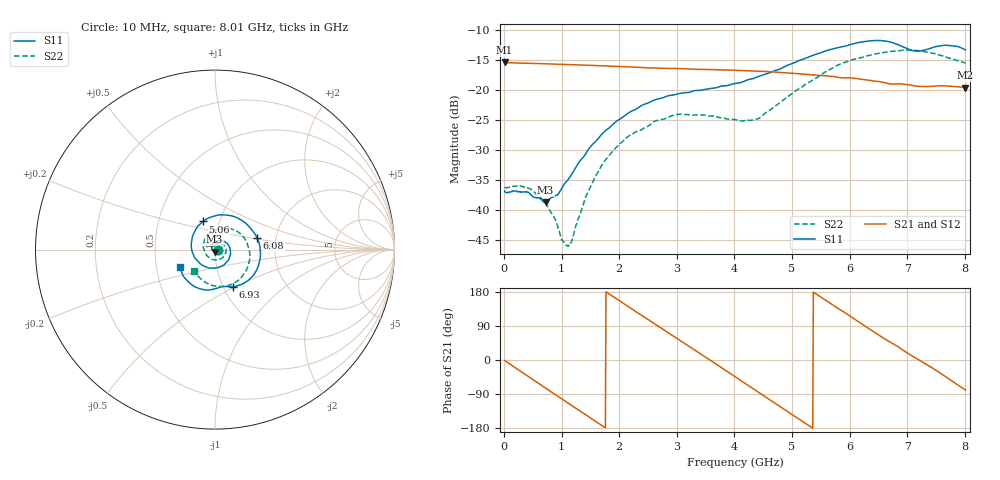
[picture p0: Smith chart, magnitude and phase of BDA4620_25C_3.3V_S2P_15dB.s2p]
!Agilent Technologies,E5071B,MY42404982,A.09.10
!Date: Wed May 06 08:51:47 2026
!Data & Calibration Information:
!Freq	S11:SOLT2(ON)	S21:SOLT2(ON)	S12:SOLT2(ON)	S22:SOLT2(ON)
# Hz S RI R 50
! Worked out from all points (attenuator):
!   801 points, 10 MHz to 8.01 GHz, reference 50 ohm
!   highest |S21| = -15.42 dB at 10 MHz (marker M1); lowest = -19.6 dB at 8.01 GHz (marker M2)
!   lowest |S11| = -38.7 dB at 720 MHz (marker M3), VSWR 1.02, Z = 49.8 - j1.13 ohm
!   |S11| at or under -10 dB: start of sweep to end of sweep
!   |S22| runs from -46.0 to -13.4 dB; largest |S21 - S12| = 0.00071
!   S11 on the Smith chart (normalised r, x): 10 MHz: 1.03, -0.00; 5.06 GHz: 0.84, +0.27; 6.08 GHz: 1.59, +0.22; 6.93 GHz: 1.11, -0.48; 8.01 GHz: 0.67, -0.13
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1e7  0.0144 -0.000941  0.1694 -0.00362  0.1696 -0.00361  0.0154 -0.000668
4.4e8  0.00887 -0.0107  0.117 -0.1188  0.1171 -0.1189  0.0135 -0.00689
7.2e8  -0.00236 -0.0114  0.0456 -0.1588  0.0456 -0.1591  0.00692 -0.00918
1.09e9  -0.0174 0.000862  -0.06 -0.1517  -0.0601 -0.1518  -0.00399 -0.0031
1.17e9  -0.0188 0.00611  -0.0805 -0.1412  -0.0807 -0.1413  -0.00547 -0.000499
1.35e9  -0.0193 0.0185  -0.1196 -0.1082  -0.1197 -0.1083  -0.00753 0.00688
1.59e9  -0.0111 0.0356  -0.1519 -0.0492  -0.1521 -0.0493  -0.00563 0.0183
1.89e9  0.0125 0.0502  -0.1542 0.0333  -0.1542 0.0334  0.00555 0.0306
2.68e9  0.0844 0.00441  0.00248 0.1522  0.00271 0.1523  0.0526 0.0185
3.4e9  0.0377 -0.0918  0.1418 0.0443  0.1421 0.0443  0.0458 -0.0415
4.01e9  -0.0773 -0.0828  0.1051 -0.1012  0.1052 -0.1015  -0.0207 -0.0528
4.42e9  -0.1296 -0.00151  0.0121 -0.1427  0.0119 -0.1428  -0.0573 -0.0105
5.06e9  -0.0666 0.1567  -0.1187 -0.069  -0.1191 -0.069  -0.0267 0.0944
5.35e9  0.0199 0.1925  -0.1337 -0.00257  -0.1339 -0.00251  0.0281 0.1166
5.68e9  0.1331 0.1727  -0.1103 0.0689  -0.1104 0.069  0.1004 0.1119
6.08e9  0.2345 0.0659  -0.0391 0.119  -0.0391 0.1192  0.1748 0.0442
6.39e9  0.249 -0.063  0.0263 0.1165  0.0262 0.1167  0.1943 -0.0326
6.68e9  0.1845 -0.1722  0.0738 0.0855  0.074 0.0857  0.1771 -0.1093
6.93e9  0.0975 -0.2064  0.1008 0.0486  0.101 0.0486  0.1367 -0.1653
7.19e9  0.0366 -0.2068  0.1072 0.0023  0.1075 0.00241  0.0677 -0.2017
7.58e9  -0.0775 -0.2199  0.0884 -0.0629  0.0887 -0.063  -0.0384 -0.1904
8.01e9  -0.1934 -0.0955  0.0197 -0.1026  0.0199 -0.1028  -0.1195 -0.1166
